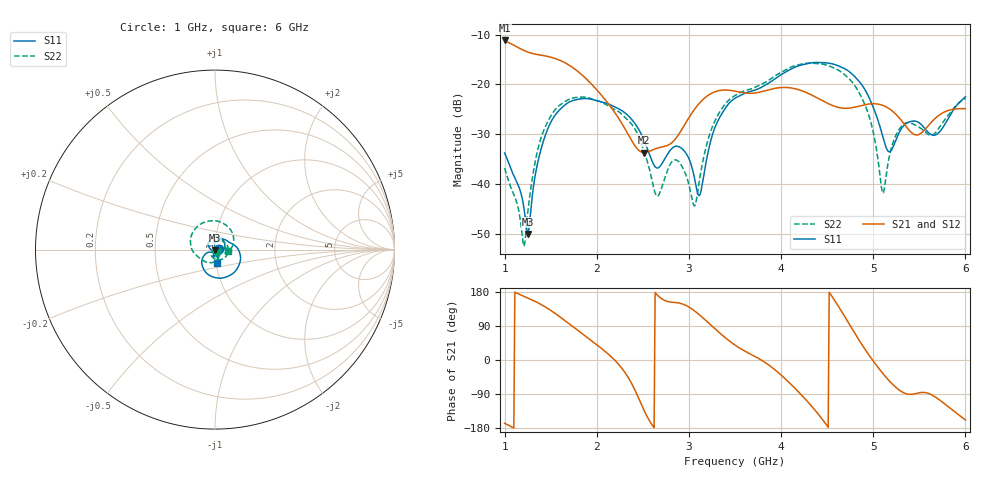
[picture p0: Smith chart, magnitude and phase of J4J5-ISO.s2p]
!Agilent Technologies,E8364B,MY43040528,A.07.50.67
!Agilent E8364B: A.07.50.67
!Date: Sunday, March 01, 2026 22:32:19
!Correction: S11(Full 2 Port(1,2))
!S21(Full 2 Port(1,2))
!S12(Full 2 Port(1,2))
!S22(Full 2 Port(1,2))
!S2P File: Measurements: S11, S21, S12, S22:
# Hz S  dB  R 50
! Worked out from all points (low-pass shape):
!   451 points, 1 GHz to 6 GHz, reference 50 ohm
!   highest |S21| = -11.18 dB at 1 GHz (marker M1); lowest = -33.6 dB at 2.511 GHz (marker M2)
!   |S21| within 3 dB of the highest: start of sweep to 1.411 GHz
!   lowest |S11| = -50.0 dB at 1.256 GHz (marker M3), VSWR 1.01, Z = 50.1 - j0.305 ohm
!   |S11| at or under -10 dB: start of sweep to end of sweep
!   |S22| runs from -52.4 to -15.7 dB; largest |S21 - S12| = 0.00095
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1e9  -33.73 15.6  -11.18 -166.9  -11.21 -166.8  -36.76 -25.9
1.2e9  -43.69 -4.4  -13.10 168.9  -13.13 168.9  -51.62 43.4
1.255556e9  -49.95 -73.2  -13.53 163.0  -13.56 163.0  -45.08 124.0
1.355556e9  -35.97 -165.7  -14.01 151.7  -14.03 151.8  -33.37 112.3
1.477778e9  -28.49 154.8  -14.43 134.5  -14.45 134.5  -27.12 81.5
1.844444e9  -22.85 74.7  -18.16 69.0  -18.19 69.0  -22.53 -11.9
2.511111e9  -31.10 -17.2  -33.64 -131.7  -33.68 -131.7  -33.27 -144.3
2.666667e9  -36.71 15.0  -32.72 169.2  -32.75 169.3  -42.33 -98.3
2.911111e9  -32.68 18.2  -29.39 149.3  -29.42 149.3  -36.02 -108.4
3.055556e9  -38.34 13.1  -25.11 130.6  -25.13 130.6  -44.35 -85.0
3.111111e9  -42.32 54.7  -23.81 119.8  -23.84 119.9  -39.55 -38.6
3.277778e9  -28.82 90.7  -21.50 83.5  -21.53 83.6  -27.46 -58.6
3.5e9  -22.76 54.9  -21.34 39.4  -21.37 39.4  -22.22 -109.1
4.344444e9  -15.63 -47.3  -22.24 -125.5  -22.27 -125.5  -15.75 109.2
4.844444e9  -19.33 -132.7  -24.35 53.1  -24.38 53.1  -21.58 -0.5
4.988889e9  -24.07 -154.2  -23.86 0.9  -23.89 1.0  -28.63 -30.8
5.1e9  -30.19 -152.1  -24.17 -34.3  -24.19 -34.4  -41.74 5.9
5.166667e9  -33.46 -123.6  -24.77 -53.1  -24.81 -53.1  -35.13 62.8
5.3e9  -29.03 -93.7  -27.10 -82.2  -27.14 -82.2  -28.51 45.0
5.466667e9  -27.39 -107.1  -30.12 -88.4  -30.15 -88.3  -28.24 16.0
5.677778e9  -30.10 -92.3  -26.72 -98.3  -26.75 -98.3  -29.60 22.0
6e9  -22.47 -82.5  -24.85 -158.1  -24.88 -158.1  -22.78 -5.4
